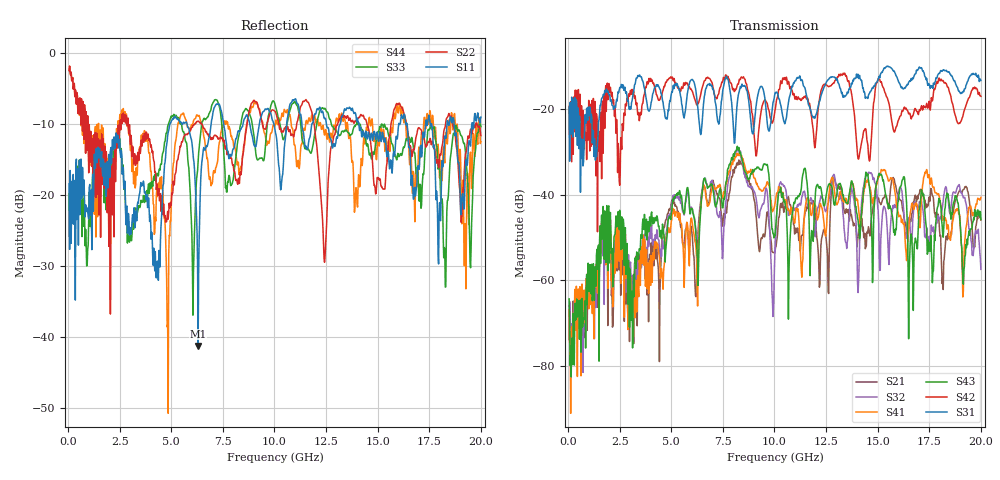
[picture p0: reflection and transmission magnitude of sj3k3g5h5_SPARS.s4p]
! FILE: E:\users\goganessyan\GBX_Backplane\FR408_backplane\1m_INBOUND_NEXT\sj3k3g5h5_SPARS.s4p
# MHZ S RI R 50.00
! FREQ  S11  S12  S13  S14
!  S21  S22  S23  S24
!  S31  S32  S33  S34
!  S41  S42  S43  S44
!  REAL  IMAG  REAL  IMAG  REAL  IMAG  REAL  IMAG
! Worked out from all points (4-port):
!   799 points, 50 MHz to 20 GHz, reference 50 ohm
!   strongest paths, dB at 50 MHz, 5.025 GHz, 10.03 GHz, 15.03 GHz, 20 GHz:
!     S31: -19.6, -16.0, -16.4, -13.3, -13.4
!     S42: -19.5, -12.9, -20.4, -13.0, -17.1
!     S43: -64.3, -43.8, -49.6, -35.8, -45.8
!     S41: -67.0, -45.8, -42.1, -35.8, -40.7
!     S32: -66.1, -41.7, -53.0, -43.9, -57.4
!     S21: -73.8, -41.4, -53.4, -41.0, -46.0
!   lowest |S11| = -41.3 dB at 6.3 GHz (marker M1), VSWR 1.02, Z = 50.1 - j0.859 ohm
!   |S11| at or under -10 dB: start of sweep to 4.938 GHz; 5.761 GHz to 6.932 GHz (1.171 GHz wide, 18.5 % of centre); 14.08 GHz to 16.02 GHz (1.938 GHz wide, 12.9 % of centre)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
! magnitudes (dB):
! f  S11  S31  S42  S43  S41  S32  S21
! 50 MHz  -18.4  -19.6  -19.5  -64.3  -67.0  -66.1  -73.8
! 4.8 GHz  -12.5  -22.4  -13.3  -49.3  -48.7  -47.5  -44.8
! 6.3 GHz  -41.3  -20.5  -18.9  -61.2  -55.8  -50.2  -48.5
! 8.2 GHz  -11.5  -18.5  -14.4  -28.7  -30.4  -29.6  -32.7
! 9.925 GHz  -9.6  -18.7  -23.0  -49.1  -43.8  -68.4  -53.5
! 10.32 GHz  -19.0  -19.6  -13.8  -39.6  -39.4  -37.4  -42.9
! 20 GHz  -9.1  -13.4  -17.1  -45.8  -40.7  -57.4  -46.0
